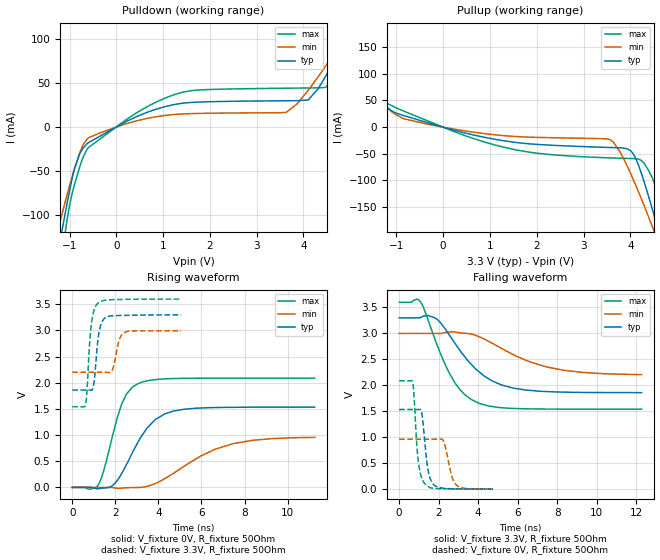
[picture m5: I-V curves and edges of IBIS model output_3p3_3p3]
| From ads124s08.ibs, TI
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|   output_3p3_3p3 Model
[Model]   output_3p3_3p3
Model_type   Output
Polarity   Non-Inverting
Vmeas = 1.65
Vref = 0
Cref = 2pF
Rref = 110
|   typ   min   max
|   (nom PVT)   (fast PVT)   (slow PVT)
C_comp   3.353e-12   3.122e-12   3.478e-12
| Where nom  PVT is Nominal Process, 3.3V, 27C
|   Fast PVT is Strong Process,  3.6V, -50C
|   Slow PVT is Weak Process,   3V, 125C
[Voltage Range]   3.3   3   3.6
|Junction Temperature
[Temperature Range]   27   125   -50
[Pullup Reference]   3.3   3   3.6
[Pulldown Reference]   0   0   0
[Power Clamp Reference]   3.3   3   3.6
[GND Clamp Reference]   0   0   0
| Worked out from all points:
|   slope of the pulldown table from 0 to 0.495 V, typ, clamps not added: 37.3 ohm
|   slope of the pullup table from 0 to 0.495 V, typ, clamps not added: 43.2 ohm
|   falling waveform, V_fixture 3.3V, R_fixture 50Ohm: 20-80 % time 1.97ns typ, 2.81ns min, 1.48ns max; typ from 3.3 V to 1.86 V
|   rising waveform, V_fixture 0V, R_fixture 50Ohm: 20-80 % time 1.34ns typ, 2.52ns min, 860ps max; typ from 0 V to 1.53 V
|   rising waveform, V_fixture 3.3V, R_fixture 50Ohm: 20-80 % time 219ps typ, 252ps min, 210ps max; typ from 1.86 V to 3.3 V
|   falling waveform, V_fixture 0V, R_fixture 50Ohm: 20-80 % time 273ps typ, 348ps min, 241ps max; typ from 1.53 V to 0.003 V
[Pulldown]
|   Voltage   I(typ)   I(min)   I(max)
-3.3V     -834.5mA   -626.7mA   -1.046A
-1.241V   -142.5mA   -116.4mA   -177.9mA
-1.158V   -117.5mA   -98.8mA    -145.1mA
-1.057V   -88.38mA   -78.2mA    -107.6mA
-897.6mV  -48.15mA   -48.01mA   -66.35mA
-704.4mV  -23.56mA   -19.74mA   -33.57mA
660mV     16.93mA    9.98mA     23.35mA
3.633V    30.09mA    16.99mA    44.42mA
4.099V    30.94mA    41.83mA    44.7mA
4.469V    57.66mA    69.23mA    45.29mA
5.089V    118.6mA    118mA      109.6mA
6.6V      274mA      240mA      307.3mA
[Pullup]
|   Voltage   I(typ)   I(min)   I(max)
-3.3V     247.2mA    200.9mA    308.8mA
-1.828V   97.21mA    83.14mA    117mA
-1.3V     46.08mA    42.76mA    52.83mA
-840mV    21.64mA    15.58mA    29.89mA
1.315V    -25.84mA   -16.09mA   -38.06mA
3.594V    -38.23mA   -24.98mA   -57.74mA
4.053V    -48.64mA   -96.28mA   -58.96mA
4.284V    -99.71mA   -145.1mA   -66.86mA
4.487V    -158.9mA   -190.7mA   -98.77mA
4.71V     -228.8mA   -243mA     -174.3mA
5.016V    -328.8mA   -317.5mA   -298.7mA
6.6V      -868.1mA   -725.7mA   -965.5mA
[Ramp]
R_load = 50
|   typ   min   max
dV/dt_r   0.920868/1.34143e-09   0.57794/2.55743e-09   1.25312/8.6004e-10
dV/dt_f   0.863979/1.97502e-09   0.480149/2.84925e-09   1.235/1.4757e-09
[Falling Waveform]
V_fixture = 3.3V
V_fixture_min = 3V
V_fixture_max = 3.6V
R_fixture = 50Ohm
|   Time   V(typ)   V(min)   V(max)
0s        3.3V       3V         3.6V
891.5ps   3.3V       3V         3.662V
1.093ns   3.308V     3V         3.603V
1.867ns   3.287V     3V         2.829V
2.811ns   2.816V     3.031V     2.055V
3.321ns   2.55V      3.003V     1.82V
4.064ns   2.254V     2.934V     1.652V
5.19ns    2.007V     2.709V     1.57V
7.464ns   1.881V     2.354V     1.544V
12.26ns   1.861V     2.207V     1.542V
[Rising Waveform]
V_fixture = 0V
V_fixture_min = 0V
V_fixture_max = 0V
R_fixture = 50Ohm
|   Time   V(typ)   V(min)   V(max)
0s        1.677nV    2.368nV    1.523nV
1.212ns   -25.81mV   -4.115uV   49.02mV
1.436ns   -12.77mV   40.97uV    285.6mV
1.867ns   34.38mV    -4.98mV    980.1mV
2.291ns   262.5mV    -14.12mV   1.588V
3.052ns   862.8mV    -2.04mV    1.983V
3.865ns   1.3V       75.42mV    2.059V
4.725ns   1.461V     275.4mV    2.08V
7.464ns   1.531V     835.6mV    2.088V
11.26ns   1.534V     956.3mV    2.088V
[Rising Waveform]
V_fixture = 3.3V
V_fixture_min = 3V
V_fixture_max = 3.6V
R_fixture = 50Ohm
|   Time   V(typ)   V(min)   V(max)
0s        1.86V      2.2V       1.542V
608.1ps   1.86V      2.2V       1.562V
891.5ps   1.858V     2.2V       3.136V
1.017ns   2.027V     2.2V       3.395V
1.212ns   2.878V     2.2V       3.528V
1.398ns   3.178V     2.2V       3.565V
1.829ns   3.278V     2.218V     3.586V
2.195ns   3.285V     2.835V     3.591V
2.443ns   3.288V     2.965V     3.593V
5.058ns   3.299V     2.995V     3.599V
[Falling Waveform]
V_fixture = 0V
V_fixture_min = 0V
V_fixture_max = 0V
R_fixture = 50Ohm
|   Time   V(typ)   V(min)   V(max)
0s        1.535V     963.2mV    2.089V
668.2ps   1.535V     963.2mV    2.078V
970.4ps   1.535V     963.2mV    533.2mV
1.137ns   1.482V     963.2mV    218.8mV
1.289ns   946mV      963.2mV    110.6mV
1.463ns   364.6mV    963.2mV    53mV
1.784ns   76.09mV    963mV      15.64mV
2.232ns   19.51mV    938mV      9.119mV
2.893ns   7.932mV    80.85mV    5.61mV
4.74ns    2.735mV    5.159mV    1.622mV
